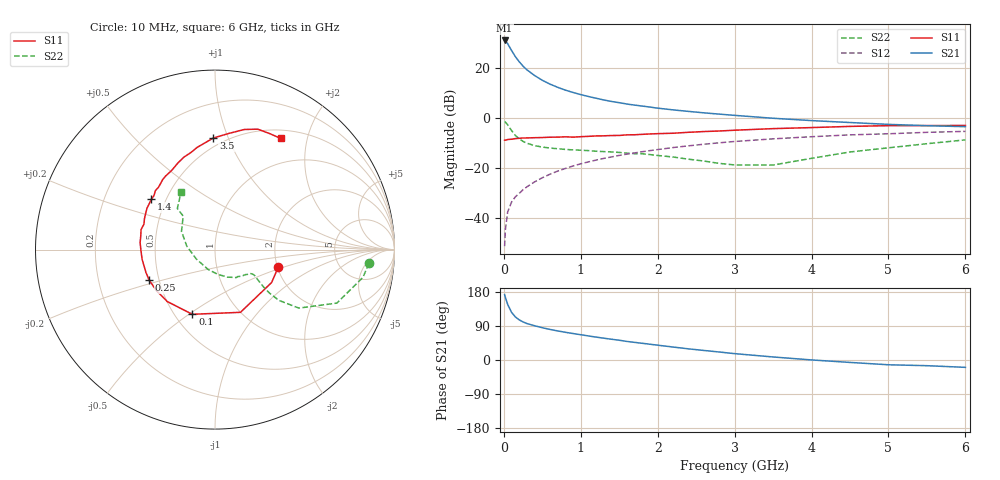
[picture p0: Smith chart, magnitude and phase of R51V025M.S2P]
! SIEMENS Small Signal Semiconductors
! BFR183
! Si NPN RF Bipolar Junction Transistor in SOT23
! VCE = 1 V  IC = 25 mA
! Common Emitter S-Parameters:  May  1996
# GHz  S  MA  R  50
!  f  S11  S21  S12  S22
! GHz  MAG  ANG  MAG  ANG  MAG  ANG  MAG  ANG
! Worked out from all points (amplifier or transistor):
!   36 points, 10 MHz to 6 GHz, reference 50 ohm
!   highest |S21| = 31.1 dB at 10 MHz (marker M1)
!   |S21| within 3 dB of that: start of sweep to 81.69 MHz
!   unconditionally stable (mu >= 1): start of sweep to 11.74 MHz; 285.9 MHz to 3.175 GHz
!   at 250 MHz: K = 0.96, MSG = 24.7 dB, |S12| = -28.5 dB
!   at 1.4 GHz: K = 1.13, MAG = 8.9 dB, |S12| = -15.4 dB
!   at 6 GHz: K = 1.00, MSG = 0.9 dB, |S12| = -5.2 dB
!   S11 on the Smith chart (normalised r, x): 10 MHz: 2.02, -0.46; 100 MHz: 0.61, -0.52; 250 MHz: 0.44, -0.18; 1.4 GHz: 0.42, +0.30; 3.5 GHz: 0.44, +0.88; 6 GHz: 0.61, +1.57
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0.01  0.366 -15.5  35.77 172.5  0.0028 81.5  0.8602 -5.1
0.02  0.3648 -30.2  35.03 165.1  0.006 77.0  0.8391 -10.6
0.05  0.3772 -67.9  30.8 146.6  0.0135 70.5  0.7416 -23.7
0.1  0.3819 -109.3  22.62 125.9  0.0212 62.8  0.5696 -34.9
0.15  0.3931 -132.6  17 113.5  0.0271 62.6  0.454 -38.5
0.2  0.3982 -145.0  13.46 105.9  0.0317 64.9  0.3893 -38.6
0.25  0.4044 -155.0  10.97 100.4  0.0376 65.5  0.3457 -37.7
0.3  0.4052 -161.7  9.285 96.2  0.0428 67.4  0.3176 -36.6
0.4  0.4097 -172.4  7.134 90.4  0.0538 69.1  0.2847 -34.7
0.5  0.4127 -179.5  5.736 85.2  0.065 69.8  0.2662 -33.3
0.6  0.419 174.7  4.805 80.7  0.0766 69.9  0.2546 -33.0
0.7  0.4206 169.5  4.152 76.7  0.0882 70.0  0.2466 -33.3
0.8  0.4268 164.8  3.646 73.1  0.0998 69.2  0.239 -34.0
1.1  0.4359 152.3  2.722 63.5  0.1348 66.9  0.2261 -37.9
1.4  0.4529 141.4  2.166 54.8  0.1694 63.7  0.2127 -43.2
1.7  0.469 132.1  1.833 46.5  0.2035 60.2  0.1967 -49.7
2.2  0.5031 118.6  1.471 34.2  0.2605 53.5  0.1687 -65.5
2.8  0.5573 103.9  1.211 21.1  0.324 45.0  0.1258 -94.2
3.5  0.6216 90.9  1.001 8.0  0.3886 34.4  0.1165 -153.1
4.5  0.6888 76.3  0.823 -6.4  0.4666 20.5  0.2126 151.4
5.5  0.7146 64.5  0.711 -15.0  0.5242 8.5  0.3108 132.5
6  0.7193 59.5  0.68 -19.4  0.5481 1.0  0.3708 120.7
